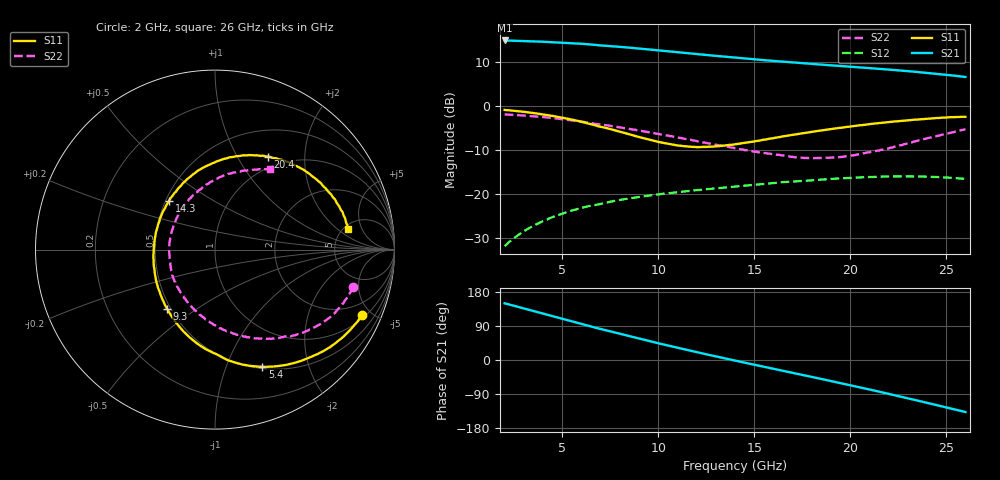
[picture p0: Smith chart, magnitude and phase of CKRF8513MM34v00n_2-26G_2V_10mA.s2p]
! CHUO DENSHI KOGYO Co.,Ltd.
! 23. June 2017
! CKRF8513MM34_RT5880
! N-channel HJ-FET
! Vds = 2 V, Id = 10 mA
# Hz S  MA  R 50
!	f	S11	S21	S12	S22
!	Hz	MAG	ANG	MAG	ANG	MAG	ANG	MAG	ANG
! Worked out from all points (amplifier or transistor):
!   241 points, 2 GHz to 26 GHz, reference 50 ohm
!   highest |S21| = 14.8 dB at 2 GHz (marker M1)
!   |S21| within 3 dB of that: start of sweep to 11.81 GHz
!   unconditionally stable (mu >= 1): 12.28 GHz to 14.4 GHz; 14.4 GHz to 14.67 GHz
!   at 6 GHz: K = 0.69, MSG = 18.6 dB, |S12| = -23.2 dB
!   at 14 GHz: K = 1.01, MAG = 14.2 dB, |S12| = -18.3 dB
!   at 26 GHz: K = 0.59, MSG = 11.6 dB, |S12| = -16.6 dB
!   lowest NFmin = 0.35 dB at 10 GHz
!   S11 on the Smith chart (normalised r, x): 2 GHz: 1.17, -4.39; 5.4 GHz: 0.52, -1.35; 9.3 GHz: 0.48, -0.39; 14.3 GHz: 0.52, +0.33; 20.4 GHz: 0.84, +1.36; 26 GHz: 5.47, +2.85
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2e9  0.8968 -24.1  5.508 149.6  0.02553 73.0  0.7972 -15.0
2.9e9  0.8592 -35.5  5.438 137.5  0.03654 66.6  0.7766 -21.6
3.8e9  0.8082 -46.8  5.353 125.2  0.04693 60.7  0.7519 -28.6
4.5e9  0.7664 -55.9  5.269 115.7  0.05451 55.8  0.7249 -34.1
5.4e9  0.704 -68.0  5.137 103.4  0.06356 49.5  0.6881 -40.9
6e9  0.6596 -76.4  5.052 95.2  0.0692 45.5  0.6588 -45.6
6.6e9  0.609 -85.0  4.935 87.0  0.07411 41.3  0.6309 -50.1
7.7e9  0.5307 -101.2  4.723 73.0  0.08323 35.6  0.5814 -58.5
8.4e9  0.4813 -112.8  4.583 64.0  0.08822 31.4  0.5497 -64.2
9.3e9  0.4244 -128.9  4.397 52.7  0.09421 26.2  0.5114 -71.6
1e10  0.3893 -142.1  4.253 44.2  0.09858 22.7  0.4807 -77.5
1.1e10  0.3546 -162.4  4.055 32.3  0.1045 17.7  0.439 -86.5
1.2e10  0.3398 176.5  3.864 20.7  0.1102 12.8  0.3982 -96.3
1.4e10  0.3658 138.4  3.516 -1.5  0.1212 3.2  0.329 -117.8
1.43e10  0.3739 133.4  3.468 -4.8  0.1228 1.8  0.32 -121.2
1.62e10  0.4378 106.0  3.201 -25.3  0.1339 -7.7  0.2775 -147.7
1.8e10  0.5062 84.8  2.983 -44.6  0.1427 -17.8  0.2557 -177.8
1.91e10  0.5486 73.3  2.867 -56.6  0.1484 -24.3  0.2585 162.3
2.04e10  0.597 60.2  2.734 -71.0  0.1537 -32.6  0.2809 137.7
2.2e10  0.6526 45.2  2.575 -89.2  0.1577 -43.9  0.3274 110.4
2.37e10  0.7046 29.0  2.395 -109.4  0.1577 -57.1  0.4113 84.3
2.6e10  0.75 8.7  2.121 -137.3  0.1478 -76.1  0.5431 55.6
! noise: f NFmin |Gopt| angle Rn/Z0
1e+10  0.35  0.286  102.3  0.09
1.05e+10  0.38  0.275  113.7  0.08
1.1e+10  0.41  0.258  121.7  0.08
1.15e+10  0.44  0.24  136.4  0.07
1.2e+10  0.46  0.23  149.8  0.06
1.25e+10  0.49  0.225  163.1  0.06
1.3e+10  0.52  0.227  178.8  0.06
1.35e+10  0.55  0.236  -166.6  0.06
1.4e+10  0.58  0.246  -153.2  0.06
1.5e+10  0.64  0.275  -129.4  0.07
